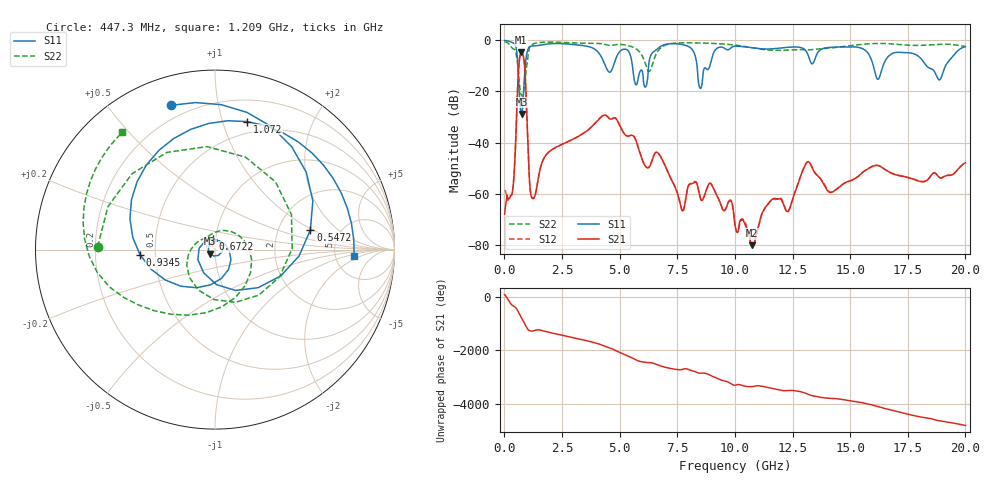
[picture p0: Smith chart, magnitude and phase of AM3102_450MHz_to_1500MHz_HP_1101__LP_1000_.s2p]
!Agilent Technologies,E8364B,MY43040894,A.07.50.67
!Agilent E8364B: A.07.50.67
!Date: Thursday, January 11, 2018 06:39:26
!Correction: S11(Full 2 Port(1,2))
!S21(Full 2 Port(1,2))
!S12(Full 2 Port(1,2))
!S22(Full 2 Port(1,2))
!S2P File: Measurements: S11, S21, S12, S22:
# Hz S  dB  R 50
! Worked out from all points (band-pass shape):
!   1601 points, 10 MHz to 20 GHz, reference 50 ohm
!   highest |S21| = -4.74 dB at 734.6 MHz (marker M1); lowest = -80.3 dB at 10.73 GHz (marker M2)
!   |S21| within 3 dB of the highest: 651.5 MHz to 852.3 MHz (200.9 MHz wide, 26.7 % of centre)
!   lowest |S11| = -28.8 dB at 747.1 MHz (marker M3), VSWR 1.08, Z = 47.2 - j2.17 ohm
!   |S11| at or under -10 dB: 5.554 GHz to 6.255 GHz (701.5 MHz wide, 11.9 % of centre); 8.358 GHz to 8.915 GHz (556.8 MHz wide, 6.45 % of centre); 18.31 GHz to 19.14 GHz (826.2 MHz wide, 4.41 % of centre)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
!   |S22| runs from -21.7 to -0.5 dB; largest |S21 - S12| = 0.0017
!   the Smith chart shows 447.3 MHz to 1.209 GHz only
!   S11 on the Smith chart (normalised r, x): 447.3 MHz: 0.13, +0.73; 547.2 MHz: 3.05, +0.94; 672.2 MHz: 0.97, +0.12; 934.5 MHz: 0.41, -0.03; 1.072 GHz: 0.39, +1.21; 1.209 GHz: 7.71, -1.31
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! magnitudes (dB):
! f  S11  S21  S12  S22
! 10 MHz  -0.1  -68.0  -58.6  -0.5
! 297.4 MHz  -0.7  -60.6  -60.7  -2.6
! 447.3 MHz  -1.5  -48.5  -48.5  -3.7
! 547.2 MHz  -5.3  -24.6  -24.5  -7.3
! 672.2 MHz  -24.3  -6.3  -6.3  -18.6
! 734.6 MHz  -28.8  -4.7  -4.7  -21.4
! 747.1 MHz  -28.8  -4.7  -4.7  -21.6
! 934.5 MHz  -7.6  -20.0  -20.1  -12.6
! 1.072 GHz  -2.7  -52.0  -52.0  -3.5
! 1.209 GHz  -2.2  -61.8  -61.8  -1.6
! 3.346 GHz  -2.0  -36.9  -36.9  -1.1
! 4.795 GHz  -8.2  -30.3  -30.3  -1.8
! 6.119 GHz  -18.3  -49.3  -49.3  -9.2
! 6.682 GHz  -3.0  -44.2  -44.2  -4.0
! 7.719 GHz  -1.7  -66.6  -67.0  -1.0
! 8.493 GHz  -18.8  -61.5  -61.4  -1.1
! 10.01 GHz  -2.3  -72.4  -72.0  -1.9
! 10.73 GHz  -2.9  -80.3  -80.0  -2.9
! 13.34 GHz  -9.2  -49.7  -49.7  -3.7
! 16.68 GHz  -6.2  -51.5  -51.5  -1.3
! 18.86 GHz  -15.5  -53.6  -53.6  -1.5
! 20 GHz  -2.5  -48.0  -47.8  -2.4
